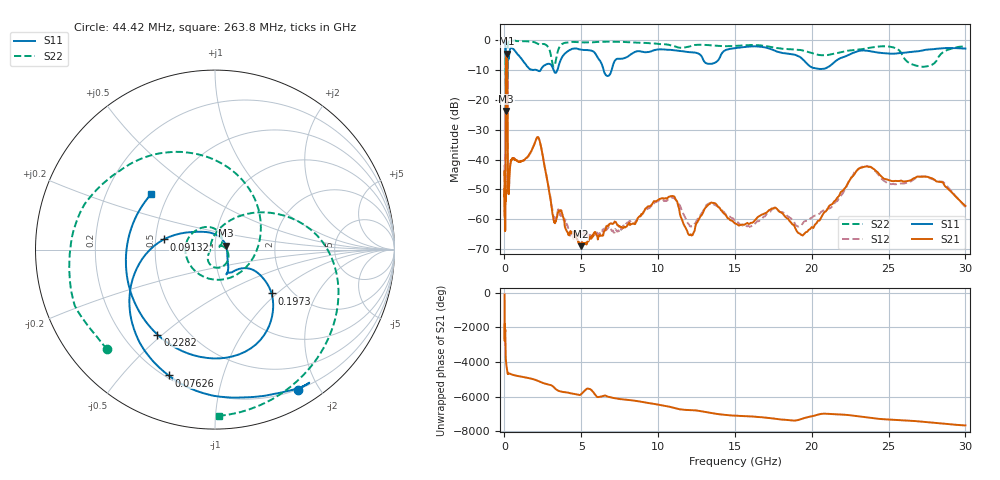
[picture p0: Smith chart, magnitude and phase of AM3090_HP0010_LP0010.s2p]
! Date/Time: Thu, Feb 28, 2019 1:55 PM
! Network Analyzer: Agilent Technologies E8364B Rev: A.07.50.67
! Sweep from 0.010 to 30.000 GHz, 1601 Points, Sweep Type: LOG
! Power Supply: 5.023 V, 0.002 A
# Hz S DB R 50
!freq MagS11 AngS11 MagS21 AngS21 MagS12 AngS12 MagS22 AngS22
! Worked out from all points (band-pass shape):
!   1601 points, 10 MHz to 30 GHz, reference 50 ohm
!   highest |S21| = -4.62 dB at 138.3 MHz (marker M1); lowest = -69.0 dB at 4.977 GHz (marker M2)
!   |S21| within 3 dB of the highest: 100.3 MHz to 184 MHz (83.65 MHz wide, 58.8 % of centre)
!   lowest |S11| = -23.8 dB at 99.43 MHz (marker M3), VSWR 1.14, Z = 56.5 + j2.4 ohm
!   |S11| at or under -10 dB: 2.054 GHz to 2.364 GHz (309.9 MHz wide, 14 % of centre); 3.197 GHz to 3.452 GHz (254.9 MHz wide, 7.67 % of centre); 6.451 GHz to 6.98 GHz (529.6 MHz wide, 7.89 % of centre)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
!   |S22| runs from -33.9 to -0.2 dB; largest |S21 - S12| = 0.013
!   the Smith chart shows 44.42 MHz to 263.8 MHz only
!   S11 on the Smith chart (normalised r, x): 44.42 MHz: 0.19, -1.74; 76.26 MHz: 0.21, -0.68; 91.32 MHz: 0.55, +0.07; 197.3 MHz: 1.59, -0.92; 228.2 MHz: 0.34, -0.48; 263.8 MHz: 0.40, +0.32
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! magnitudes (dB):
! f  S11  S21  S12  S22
! 10 MHz  -0.2  -45.1  -51.0  -0.5
! 38.04 MHz  -0.5  -60.6  -62.9  -1.4
! 44.42 MHz  -0.8  -56.4  -59.3  -1.7
! 76.26 MHz  -2.5  -44.9  -44.8  -4.9
! 91.32 MHz  -10.7  -15.2  -15.2  -15.4
! 99.43 MHz  -23.8  -8.0  -7.9  -15.9
! 126.4 MHz  -16.5  -4.8  -4.8  -33.7
! 138.3 MHz  -16.4  -4.6  -4.6  -25.6
! 144.7 MHz  -16.1  -4.7  -4.6  -21.8
! 177.7 MHz  -14.1  -6.5  -6.4  -31.3
! 197.3 MHz  -8.0  -15.0  -15.0  -11.4
! 228.2 MHz  -4.9  -49.5  -50.8  -1.6
! 263.8 MHz  -6.5  -51.3  -50.9  -0.7
! 550.5 MHz  -3.0  -39.7  -39.7  -0.3
! 2.084 GHz  -10.0  -33.0  -33.0  -1.0
! 3.204 GHz  -10.1  -60.4  -59.4  -8.8
! 4.977 GHz  -3.2  -69.0  -64.8  -0.8
! 7.926 GHz  -5.8  -62.5  -61.4  -0.7
! 10.65 GHz  -3.3  -52.6  -53.5  -1.6
! 19.7 GHz  -8.0  -64.2  -60.5  -3.9
! 23.48 GHz  -3.5  -42.4  -42.2  -2.9
! 30 GHz  -2.9  -55.5  -56.0  -2.2
